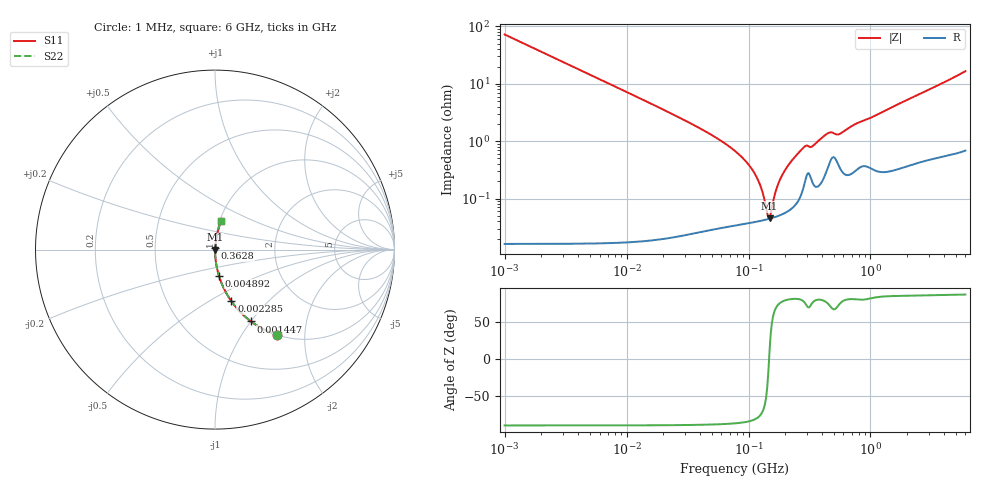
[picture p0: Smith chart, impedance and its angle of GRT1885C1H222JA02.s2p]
!Murata Part Number: GRT1885C1H222JA02
!These Parameters are Measured in Series Mode Connection
!Data Generated on Jun 19, 2026
!  o--ll--o
!Port1  Port2
!  o------o
!Operation Temp=25[degC], DC Bias Voltage=0[V]
!Freq. Start=1000[kHz] Stop=6[GHz] 401[Steps]
# Hz S RI R 50
!Freq.(Hz) S11(Real) S11(Imag) S21(Real) S21(Imag) S12(Real) S12(Imag) S22(Real) S22(Imag)
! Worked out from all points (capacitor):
!   401 points, 1 MHz to 6 GHz, reference 50 ohm
!   read as one part in series: C = 2.2 nF near 1.044 MHz
!   lowest |Z| = 45.4 mohm at 148.7 MHz (marker M1)
!   series resonance near 147.4 MHz, so ESL is about 530 pH
!   S11 on the Smith chart (normalised r, x): 1 MHz: 1.00, -1.45; 1.447 MHz: 1.00, -1.00; 2.285 MHz: 1.00, -0.63; 4.892 MHz: 1.00, -0.30; 362.8 MHz: 1.00, +0.02; 6 GHz: 1.01, +0.33
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1000000  0.3439 -0.4749  0.6561 0.4749  0.6561 0.4749  0.3439 -0.4749
1447343  0.2002 -0.4  0.7998 0.4  0.7998 0.4  0.2002 -0.4
2285201  0.0913 -0.2878  0.9087 0.2878  0.9087 0.2878  0.0913 -0.2878
4293785  0.0277 -0.1638  0.9723 0.1638  0.9723 0.1638  0.0277 -0.1638
4892295  0.0215 -0.1446  0.9785 0.1446  0.9785 0.1446  0.0215 -0.1446
1.843659e7  0.00168 -0.0385  0.9983 0.0385  0.9983 0.0385  0.00168 -0.0385
4.596069e7  0.000475 -0.0141  0.9995 0.0141  0.9995 0.0141  0.000475 -0.0141
7.745967e7  0.000383 -0.00673  0.9996 0.00673  0.9996 0.00673  0.000383 -0.00673
9.627852e7  0.000385 -0.0043  0.9996 0.0043  0.9996 0.0043  0.000385 -0.0043
1.145757e8  0.000398 -0.0025  0.9996 0.0025  0.9996 0.0025  0.000398 -0.0025
1.277378e8  0.000413 -0.00141  0.9996 0.00141  0.9996 0.00141  0.000413 -0.00141
1.424119e8  0.000434 -0.000339  0.9996 0.000339  0.9996 0.000339  0.000434 -0.000339
1.487431e8  0.000445 9.01e-05  0.9996 -9.01e-05  0.9996 -9.01e-05  0.000445 9.01e-05
1.732027e8  0.000495 0.00161  0.9995 -0.00161  0.9995 -0.00161  0.000495 0.00161
2.016844e8  0.000579 0.00321  0.9994 -0.00321  0.9994 -0.00321  0.000579 0.00321
2.794814e8  0.00149 0.00742  0.9985 -0.00742  0.9985 -0.00742  0.00149 0.00742
3.325952e8  0.00201 0.00781  0.998 -0.00781  0.998 -0.00781  0.00201 0.00781
3.628252e8  0.00168 0.00938  0.9983 -0.00938  0.9983 -0.00938  0.00168 0.00938
4.509737e8  0.00381 0.0133  0.9962 -0.0133  0.9962 -0.0133  0.00381 0.0133
5.60538e8  0.00358 0.0129  0.9964 -0.0129  0.9964 -0.0129  0.00358 0.0129
1.428092e9  0.00431 0.0368  0.9957 -0.0368  0.9957 -0.0368  0.00431 0.0368
6e9  0.0331 0.1594  0.9669 -0.1594  0.9669 -0.1594  0.0331 0.1594
